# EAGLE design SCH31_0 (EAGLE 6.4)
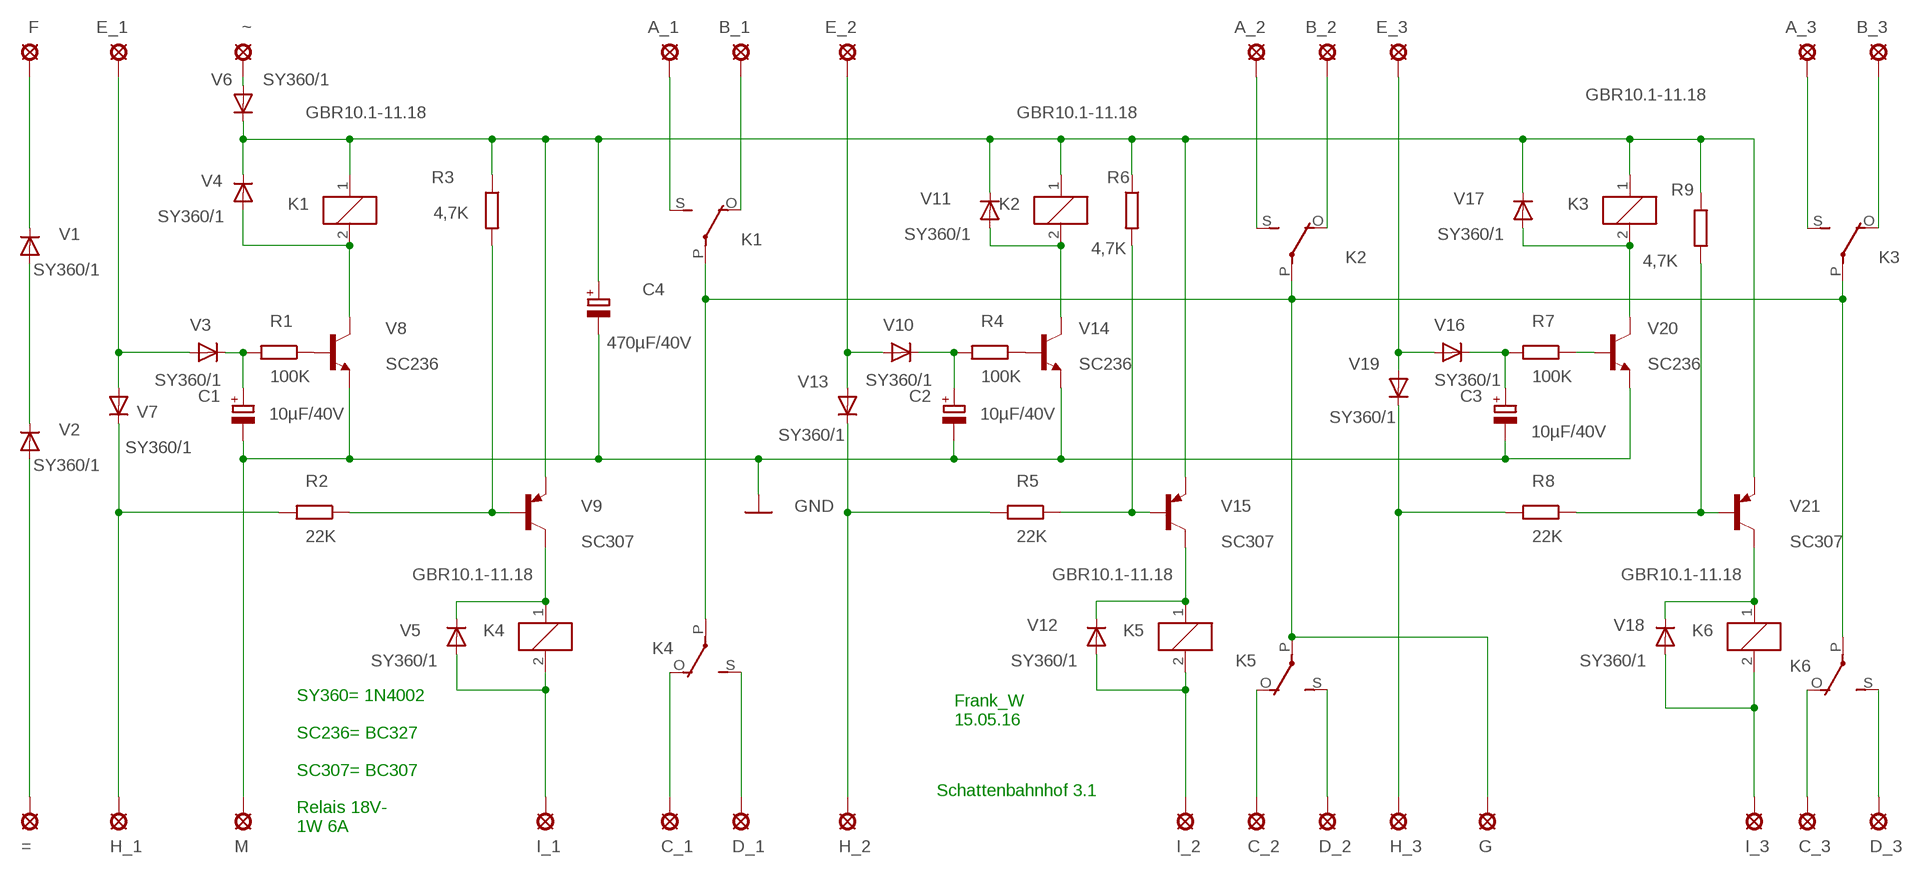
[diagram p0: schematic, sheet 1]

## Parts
=  LSP10  [LSP10]
A_1  LSP10  [LSP10]
A_2  LSP10  [LSP10]
A_3  LSP10  [LSP10]
B_1  LSP10  [LSP10]
B_2  LSP10  [LSP10]
B_3  LSP10  [LSP10]
C1  10µF/40V  CPOL-EUE5-5  [E5-5]
C2  10µF/40V  CPOL-EUE5-5  [E5-5]
C3  10µF/40V  CPOL-EUE5-5  [E5-5]
C4  470µF/40V  CPOL-EUE22-9AXIAL  [E22-9]
C_1  LSP10  [LSP10]
C_2  LSP10  [LSP10]
C_3  LSP10  [LSP10]
D_1  LSP10  [LSP10]
D_2  LSP10  [LSP10]
D_3  LSP10  [LSP10]
E_1  LSP10  [LSP10]
E_2  LSP10  [LSP10]
E_3  LSP10  [LSP10]
F  LSP10  [LSP10]
G  LSP10  [LSP10]
H_1  LSP10  [LSP10]
H_2  LSP10  [LSP10]
H_3  LSP10  [LSP10]
I_1  LSP10  [LSP10]
I_2  LSP10  [LSP10]
I_3  LSP10  [LSP10]
K1  GBR10.1-11.18  G2R  [G2R]
K2  GBR10.1-11.18  G2R  [G2R]
K3  GBR10.1-11.18  G2R  [G2R]
K4  GBR10.1-11.18  G2R  [G2R]
K5  GBR10.1-11.18  G2R  [G2R]
K6  GBR10.1-11.18  G2R  [G2R]
M  LSP10  [LSP10]
R1  100K  R-EU_0207/12  [0207/12]
R2  22K  R-EU_0207/12  [0207/12]
R3  4,7K  R-EU_0207/12  [0207/12]
R4  100K  R-EU_0207/12  [0207/12]
R5  22K  R-EU_0207/12  [0207/12]
R6  4,7K  R-EU_0207/12  [0207/12]
R7  100K  R-EU_0207/12  [0207/12]
R8  22K  R-EU_0207/12  [0207/12]
R9  4,7K  R-EU_0207/12  [0207/12]
V1  SY360/1  1N4004  [DO41-10]
V2  SY360/1  1N4004  [DO41-10]
V3  SY360/1  1N4004  [DO41-10]
V4  SY360/1  1N4004  [DO41-10]
V5  SY360/1  1N4004  [DO41-10]
V6  SY360/1  1N4004  [DO41-10]
V7  SY360/1  1N4004  [DO41-10]
V8  SC236  BC449  [TO92-EBC]
V9  SC307  BC448  [TO92-EBC]
V10  SY360/1  1N4004  [DO41-10]
V11  SY360/1  1N4004  [DO41-10]
V12  SY360/1  1N4004  [DO41-10]
V13  SY360/1  1N4004  [DO41-10]
V14  SC236  BC449  [TO92-EBC]
V15  SC307  BC448  [TO92-EBC]
V16  SY360/1  1N4004  [DO41-10]
V17  SY360/1  1N4004  [DO41-10]
V18  SY360/1  1N4004  [DO41-10]
V19  SY360/1  1N4004  [DO41-10]
V20  SC236  BC449  [TO92-EBC]
V21  SC307  BC448  [TO92-EBC]
~  LSP10  [LSP10]

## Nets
GND: C1.- C2.- C3.- C4.- M.MP V8.E V14.E V20.E
N$1: =.MP V2.A
N$2: V1.A V2.C
N$3: R1.1 V8.B
N$4: F.MP V1.C
N$5: E_1.MP V3.A V7.A
N$6: C1.+ R1.2 V3.C
N$7: R4.1 V14.B
N$8: K1.2 V4.A V8.C
N$9: V6.A ~.MP
N$10: C4.+ K1.1 K2.1 K3.1 R3.1 R6.1 R9.1 V4.C V6.C V9.E V11.C V15.E V17.C V21.E
N$11: H_1.MP R2.2 V7.C
N$12: R2.1 R3.2 V9.B
N$14: K5.1 V12.C V15.C
N$15: G.MP K1.P(2:P) K2.P(2:P) K3.P(2:P) K4.P(2:P) K5.P(2:P) K6.P(2:P)
N$16: B_1.MP K1.O(2:O)
N$17: A_1.MP K1.S(2:S)
N$18: C_1.MP K4.O(2:O)
N$19: D_1.MP K4.S(2:S)
N$20: H_2.MP R5.2 V13.C
N$21: E_2.MP V10.A V13.A
N$22: K2.2 V11.A V14.C
N$23: B_2.MP K2.O(2:O)
N$24: C2.+ R4.2 V10.C
N$25: A_2.MP K2.S(2:S)
N$26: R5.1 R6.2 V15.B
N$27: A_3.MP K3.S(2:S)
N$28: B_3.MP K3.O(2:O)
N$29: C_2.MP K5.O(2:O)
N$30: K4.1 V5.C V9.C
N$31: I_2.MP K5.2 V12.A
N$32: D_2.MP K5.S(2:S)
N$33: E_3.MP V16.A V19.A
N$34: R7.1 V20.B
N$35: C3.+ R7.2 V16.C
N$36: K3.2 V17.A V20.C
N$37: R8.1 R9.2 V21.B
N$38: I_1.MP K4.2 V5.A
N$39: K6.1 V18.C V21.C
N$40: H_3.MP R8.2 V19.C
N$41: I_3.MP K6.2 V18.A
N$44: C_3.MP K6.O(2:O)
N$45: D_3.MP K6.S(2:S)

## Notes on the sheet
- Frank_W
  15.05.16
- Schattenbahnhof 3.1
- SY360= 1N4002
  
  SC236= BC327
  
  SC307= BC307
  
  Relais 18V-
  1W 6A

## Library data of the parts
= A_1-A_3 B_1-B_3 C_1-C_3 D_1-D_3 E_1-E_3 F G H_1-H_3 I_1-I_3 M ~ = solpad:LSP10: SOLDER PAD
C1-C4 = rcl:CPOL-EU: POLARIZED CAPACITOR, European symbol
K1-K6 = relay:G2R: RELAY 1 x switch, Omron; OC_FARNELL: 1569185; OC_NEWARK: unknown
R1-R9 = rcl:R-EU_: RESISTOR, European symbol
V1-V7 V10-V13 V16-V19 = diode:1N4004: DIODE
V8 V14 V20 = transistor-npn:BC449*: NPN Transistor
V9 V15 V21 = transistor-pnp:BC448*: PNP Transistror

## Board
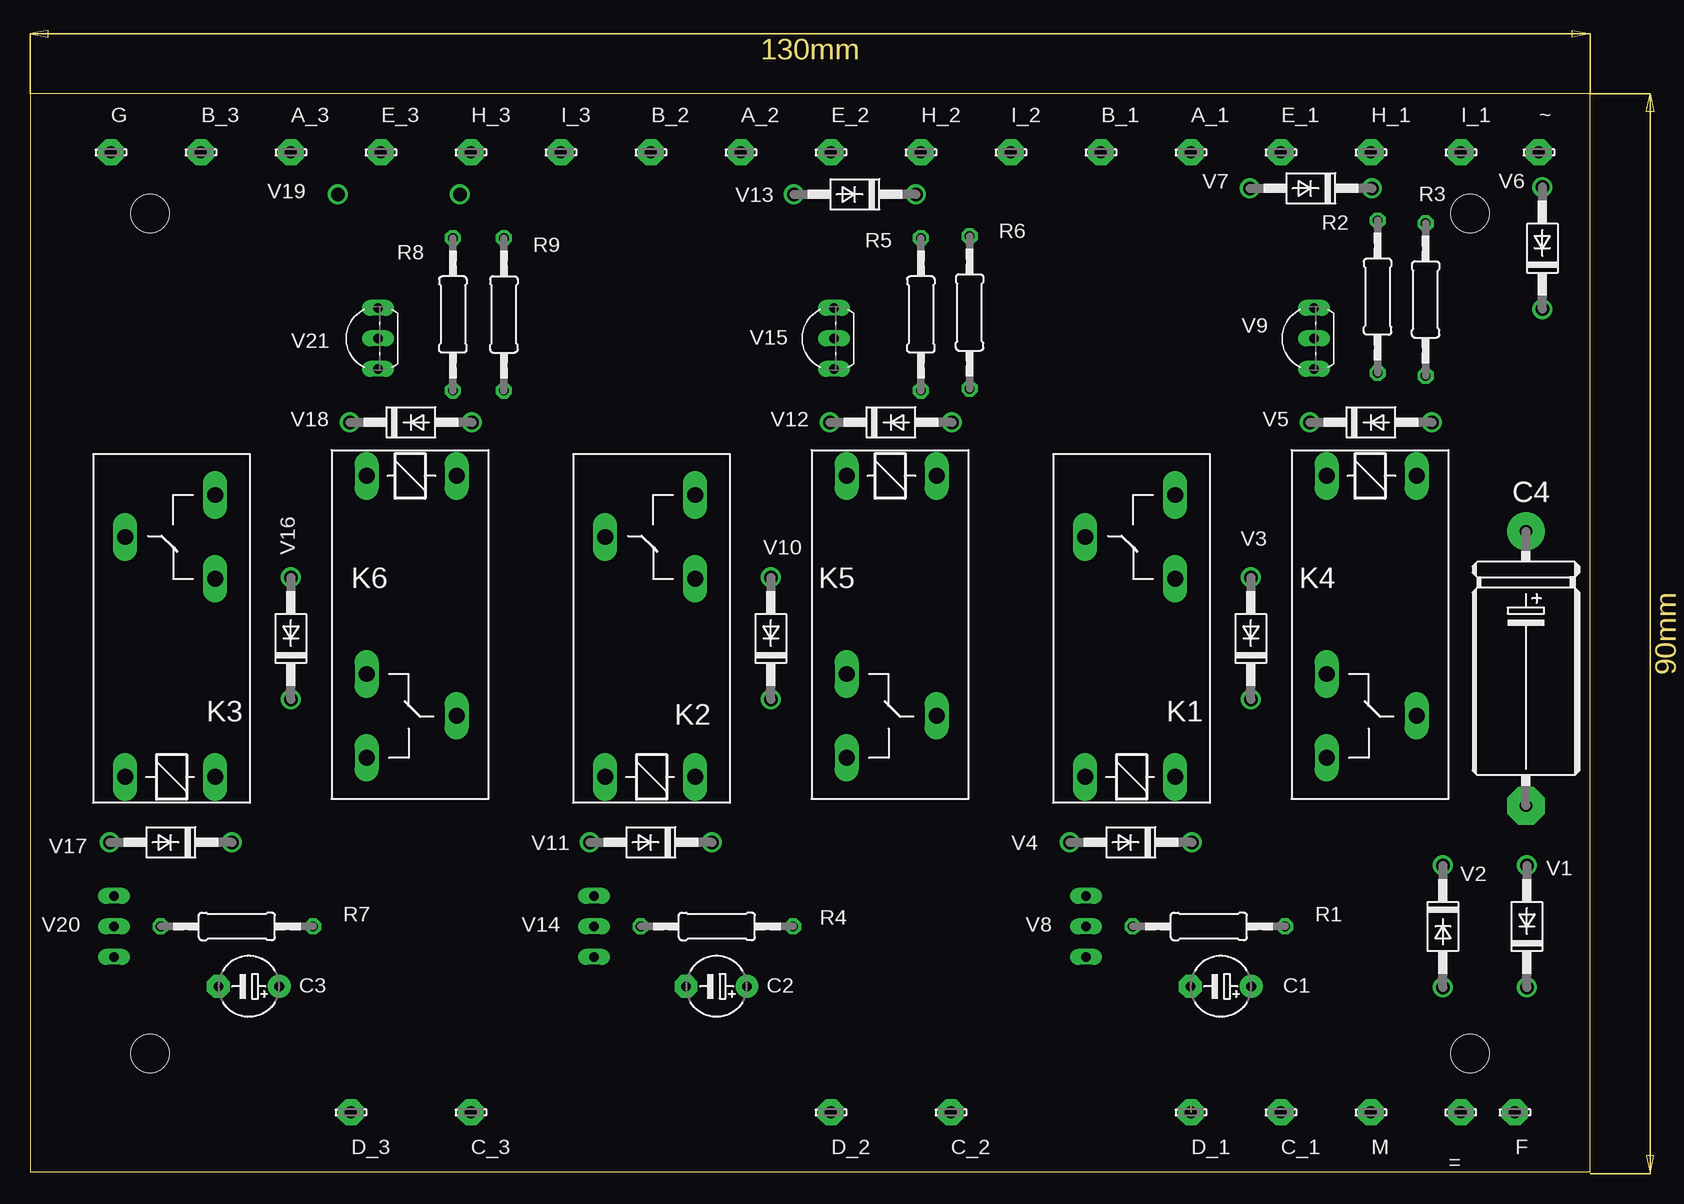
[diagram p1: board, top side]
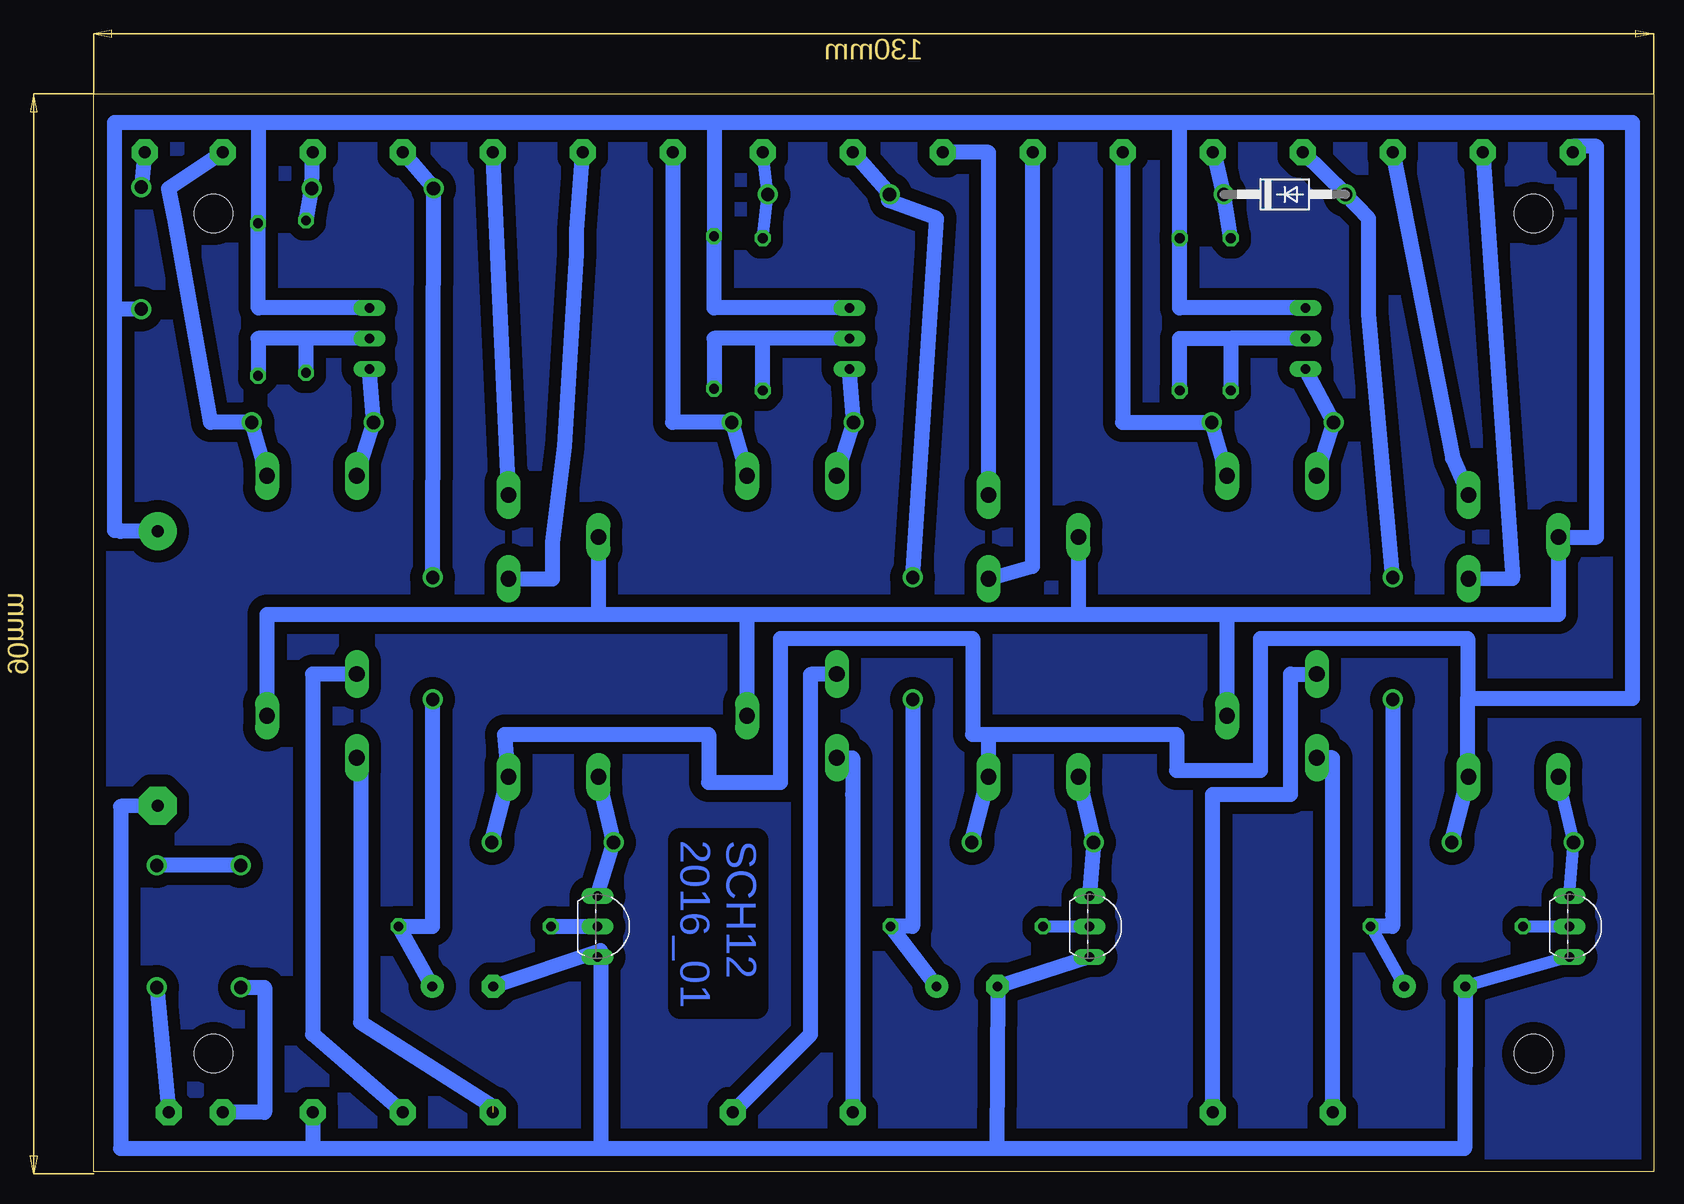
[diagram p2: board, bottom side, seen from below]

Size 135.3 x 95.3 mm. Coordinates in mm from the lower left corner, seen from the top.
Outline: 0,90 0,0.16 130,0.16 130,90 0,90
Copper layers (1*16): Top 0.035mm / dielectric 1.5mm / Bottom 0.035mm
Design rules "default *": minimum track width 20mil, minimum drill 24mil, track to track 8mil, track to pad 8mil, pad to pad 8mil, via to via 8mil, smd to smd 8mil, copper to edge 40mil, drill to drill 8mil, minimum pad ring 10mil, minimum via ring 8mil, stop-mask expansion 4mil, vias tented up to drill 0mil, thermal gap 20mil
Holes 3.2 mm at 120,10 10,10 10,80 120,80

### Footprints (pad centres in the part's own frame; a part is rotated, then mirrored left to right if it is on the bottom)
LSP10 = drill 1.016 pad 2.159 octagon: MP 0,0
E5-5 = drill 0.813 pad 1.905: + -2.54,0 | drill 0.813 pad 1.905 octagon: - 2.54,0
E22-9 = drill 1.016 pad 3.15: + -11.43,0 | drill 1.016 pad 3.15 octagon: - 11.43,0
G2R = drill 1.321 long: 1 -2.54,-3.683; 2 -2.54,3.81; O 13.97,-3.683; P 17.45,3.81; S 20.955,-3.683
0207/12 = drill 0.813 octagon: 1 -6.35,0; 2 6.35,0
DO41-10 = drill 1.118: A 5.08,0; C -5.08,0
TO92-EBC = drill 0.813 long: B 0,-1.27; C -2.54,-1.27; E 2.54,-1.27

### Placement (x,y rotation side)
=  119.24,5.1 180 top
A_1  96.74,85.1 0 top
A_2  59.24,85.1 0 top
A_3  21.74,85.1 0 top
B_1  89.24,85.1 0 top
B_2  51.74,85.1 0 top
B_3  14.24,85.1 0 top
C1  99.24,15.6 180 top
C2  57.21,15.6 180 top
C3  18.24,15.6 180 top
C4  124.66,42.09 270 top
C_1  104.24,5.1 0 top
C_2  76.74,5.1 0 top
C_3  36.74,5.1 0 top
D_1  96.74,5.1 0 top
D_2  66.74,5.1 0 top
D_3  26.74,5.1 0 top
E_1  104.24,85.1 0 top
E_2  66.74,85.1 0 top
E_3  29.24,85.1 0 top
F  123.74,5.1 0 top
G  6.74,85.1 0 top
H_1  111.74,85.1 0 top
H_2  74.24,85.1 0 top
H_3  36.74,85.1 0 top
I_1  119.24,85.1 0 top
I_2  81.74,85.1 0 top
I_3  44.24,85.1 0 top
K1  91.74,35.6 90 top
K2  51.74,35.6 90 top
K3  11.74,35.6 90 top
K4  111.74,55.6 270 top
K5  71.74,55.6 270 top
K6  31.74,55.6 270 top
M  111.74,5.1 0 top
R1  98.24,20.6 0 top
R2  112.3,73.08 90 top
R3  116.3,72.84 270 top
R4  57.24,20.6 0 top
R5  74.24,71.6 90 top
R6  78.3,71.76 270 top
R7  17.24,20.6 0 top
R8  35.24,71.6 90 top
R9  39.49,71.6 270 top
V1  124.74,20.6 90 top
V2  117.74,20.6 270 top
V3  101.74,44.6 90 top
V4  91.74,27.6 180 top
V5  111.74,62.6 0 top
V6  126.03,77.12 90 top
V7  106.74,82.1 180 top
V8  86.74,20.6 270 bottom
V9  105.74,69.6 90 top
V10  61.74,44.6 90 top
V11  51.74,27.6 180 top
V12  71.74,62.6 0 top
V13  68.74,81.6 180 top
V14  45.74,20.6 270 bottom
V15  65.74,69.6 90 top
V16  21.74,44.6 90 top
V17  11.74,27.6 180 top
V18  31.74,62.6 0 top
V19  30.74,81.6 0 bottom
V20  5.74,20.6 270 bottom
V21  27.74,69.6 90 top
~  125.74,85.1 0 top

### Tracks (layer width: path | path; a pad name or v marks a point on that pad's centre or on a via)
GND
  Bottom 1.016: V20.E C3.-
  Bottom 1.27: C1.- 87.74,18.6 | 87.74,18.6 V8.E | C4.- 127.74,30.6 127.74,2.1 111.74,2.1 | 111.74,2.1 87.74,2.1 | 87.74,2.1 54.74,2.1 | 54.74,2.1 15.74,2.1 C3.- | 87.74,18.6 87.74,2.1 | 54.74,2.1 C2.- V14.E | M.MP 111.74,2.1
N$1
  Bottom 1.27: V2.A 115.74,15.52 115.74,5.1 =.MP
N$2
  Bottom 1.27: V2.C V1.A
N$3
  Bottom 1.27: R1.1 V8.B
N$4
  Bottom 1.27: V1.C F.MP
N$5
  Bottom 1.27: V3.A V7.A E_1.MP
N$6
  Bottom 1.27: C1.+ R1.2 101.74,20.6 101.74,21.6 V3.C
N$7
  Bottom 1.016: R4.1 V14.B
N$8
  Bottom 1.27: V8.C V4.A K1.2
N$9
  Bottom 1.27: ~.MP V6.A
N$10
  Bottom 1.27: V4.C K1.1 95.74,36.6 78.74,36.6 78.74,32.6 72.74,32.6 72.74,44.6 56.74,44.6 56.74,36.6 55.42,36.6 | V21.E 39.49,72.14 R9.1 39.49,87.6 | V15.E 78.3,72.14 R6.1 78.24,78.55 78.24,87.6 | V9.E 116.24,72.14 116.3,72.2 R3.1 116.24,79.75 116.24,87.6 | 116.24,87.6 78.24,87.6 | 78.24,87.6 39.49,87.6 | 39.49,87.6 1.74,87.6 1.74,39.6 15.49,39.6 | 15.49,39.6 15.49,33.38 K3.1 V17.C | 55.42,36.6 39.74,36.6 39.74,33.6 32.74,33.6 32.74,44.6 15.49,44.6 15.49,39.6 | V11.C K2.1 55.42,36.6 | 116.24,87.6 128.24,87.6 128.24,72.6 128.24,72.04 | C4.+ 127.74,53.52 127.74,53.6 128.24,53.6 128.24,72.04 | V6.C 128.24,72.04
N$11
  Bottom 1.27: R2.2 V7.C H_1.MP
N$12
  Bottom 1.27: V9.B 112.3,69.6 | 112.3,69.6 116.3,69.6 R3.2 | R2.1 112.3,69.6
N$13
  pour Bottom (isolate 1.016): 0.74,89.6 129.74,89.6 129.74,0.6 0.74,0.6
N$14
  Bottom 1.27: K5.1 V12.C V15.C
N$15
  Bottom 1.27: K4.P 115.55,46.6 87.93,46.6 | 87.93,46.6 75.55,46.6 | 75.55,46.6 47.93,46.6 | 47.93,46.6 35.55,46.6 | 35.55,46.6 7.93,46.6 K3.P 4.74,53.05 4.74,85.6 6.74,85.6 G.MP | K1.P 87.93,46.6 | K5.P 75.55,46.6 | K2.P 47.93,46.6 | K6.P 35.55,46.6
N$16
  Bottom 1.27: K1.O 91.74,49.57 91.74,52.6 90.74,60.6 89.74,76.6 89.74,78.6 B_1.MP
N$17
  Bottom 1.27: K1.S 96.74,85.6 A_1.MP
N$18
  Bottom 1.27: K4.O 111.74,41.63 111.74,11.6 C_1.MP
N$19  (1 unrouted)
  Bottom 1.27: K4.S 107.74,34.65 107.74,12.6 96.74,5.6
N$20
  Bottom 1.016: R5.2 V13.C H_2.MP
N$21
  Bottom 1.27: V10.A 59.74,79.6 63.74,81.08 V13.A E_2.MP
N$22
  Bottom 1.27: K2.2 V11.A V14.C
N$23
  Bottom 1.27: K2.O 51.74,50.6 B_2.MP
N$24
  Bottom 1.27: C2.+ R4.2 61.74,20.6 V10.C 61.74,39.6
N$25
  Bottom 1.27: K2.S 55.42,85.1 A_2.MP
N$26
  Bottom 1.27: V15.B 74.24,69.6 | 74.24,69.6 78.3,69.6 R6.2 | R5.1 74.24,69.6
N$27
  Bottom 1.27: A_3.MP 16.74,59.6 K3.S
N$28
  Bottom 1.27: K3.O 11.74,49.6 B_3.MP
N$29
  Bottom 1.27: C_2.MP 70.24,11.6 70.24,41.6 K5.O
N$30
  Bottom 1.27: K4.1 V5.C V9.C
N$31
  Bottom 1.27: I_2.MP 81.74,62.6 V12.A K5.2
N$32
  Bottom 1.27: K5.S 66.74,34.65 66.74,31.6 D_2.MP
N$33
  Bottom 1.27: E_3.MP V19.A 23.74,79.6 23.74,71.6 V16.A
N$34
  Bottom 1.016: R7.1 V20.B
N$35
  Bottom 1.016: C3.+ R7.2
  Bottom 1.27: V16.C 21.74,21.6 21.74,20.6 R7.2
N$36
  Bottom 1.016: V20.C V17.A K3.2
N$37
  Bottom 1.27: V21.B 35.24,69.6 | 35.24,69.6 R8.1 | R9.2 39.49,69.6 35.24,69.6
N$38
  Bottom 1.27: K4.2 V5.A 120.24,62.6 123.24,79.6 123.74,82.1 I_1.MP
N$39
  Bottom 1.27: K6.1 V18.C V21.C
N$40
  Bottom 1.27: H_3.MP 36.74,85.6 V19.C R8.2
N$41
  Bottom 1.27: K6.2 V18.A 44.24,62.6 I_3.MP
N$44
  Bottom 1.27: K6.O 30.24,41.63 30.24,31.6 36.74,31.6 C_3.MP
N$45
  Bottom 1.27: D_3.MP 26.74,33.6 26.74,34.65 K6.S

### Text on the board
Bottom: SCH12 / 2016_01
